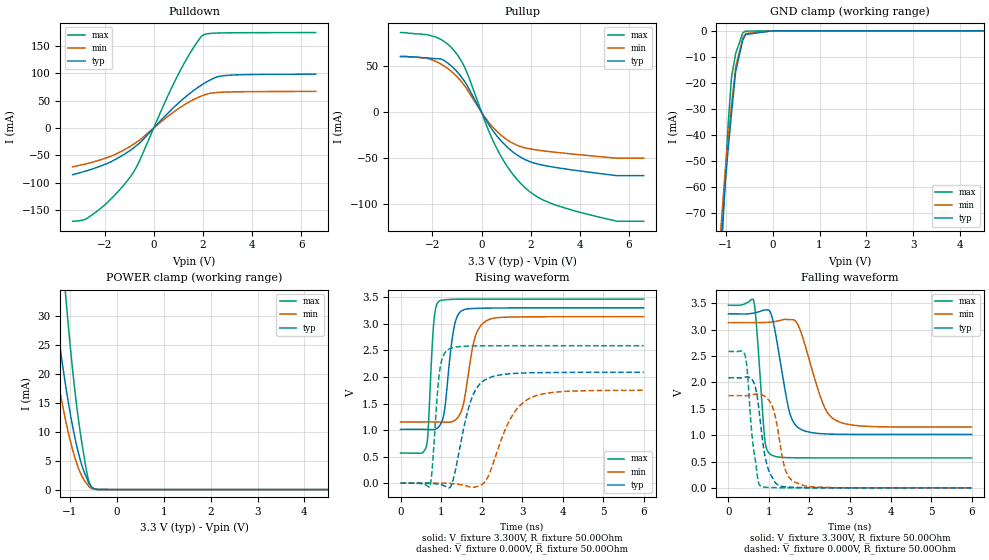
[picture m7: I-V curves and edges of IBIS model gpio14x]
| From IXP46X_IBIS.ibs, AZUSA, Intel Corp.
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[Model]   gpio14x
Model_type   I/O
Vinl = 800.000mV
Vinh = 2.000V
Vmeas = 1.500V
Cref = 0.000F
|   typ   min   max
C_comp   3.000pF   2.700pF   3.300pF
[Voltage Range]   3.300V   3.135V   3.465V
[Temperature Range]   25.0   110.0   -40.0
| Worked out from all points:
|   slope of the pulldown table from 0 to 0.495 V, typ, clamps not added: 21.2 ohm
|   slope of the pullup table from 0 to 0.495 V, typ, clamps not added: 23.4 ohm
|   POWER clamp passes 1 mA (typ) near -0.59 V on its own axis
|   falling waveform, V_fixture 3.300V, R_fixture 50.00Ohm: 20-80 % time 314ps typ, 480ps min, 160ps max; typ from 3.3 V to 1.01 V
|   rising waveform, V_fixture 3.300V, R_fixture 50.00Ohm: 20-80 % time 197ps typ, 269ps min, 114ps max; typ from 1.01 V to 3.3 V
|   rising waveform, V_fixture 0.000V, R_fixture 50.00Ohm: 20-80 % time 396ps typ, 599ps min, 153ps max; typ from 0 V to 2.09 V
|   falling waveform, V_fixture 0.000V, R_fixture 50.00Ohm: 20-80 % time 236ps typ, 261ps min, 185ps max; typ from 2.09 V to 0 V
[Pulldown]
|   Voltage   I(typ)   I(min)   I(max)
-3.3V     -85.26mA   -70.8mA    -170.3mA
-2.8V     -79.09mA   -65.87mA   -166.9mA
-2.265V   -71.22mA   -59.42mA   -150.5mA
-1.585V   -57.94mA   -48.61mA   -122.4mA
-920mV    -39.75mA   -32.53mA   -87.22mA
-600mV    -28.51mA   -22.88mA   -62.16mA
370mV     17.69mA    13.98mA    38.37mA
940mV     42.72mA    33.25mA    92.55mA
1.535V    65.34mA    49.72mA    140.7mA
1.99V     79.66mA    59.11mA    169mA
2.875V    95.55mA    65.49mA    173.5mA
6.595V    98.21mA    66.77mA    174.1mA
[GND Clamp]
|   Voltage   I(typ)   I(min)   I(max)
-3.3V     -1.837A    -1.782A    -2.189A
-1.105V   -83.62mA   -76.71mA   -91.97mA
-1.01V    -58.95mA   -53.8mA    -56.61mA
-950mV    -46.12mA   -41.91mA   -36.62mA
-875mV    -31.66mA   -28.69mA   -17.73mA
-785mV    -15.53mA   -13.65mA   -8.617mA
-635mV    -3.543mA   -2.725mA   -731.7uA
-575mV    -1.513mA   -1.109mA   -135.3uA
0V        -56.84nA   -17.58nA   -65.5pA
6.595V    0A         0A         0A
[Pullup]
|   Voltage   I(typ)   I(min)   I(max)
-3.3V     60.91mA    60.82mA    86.88mA
-1.9V     58.57mA    55.85mA    82.23mA
-1.595V   57.58mA    51.65mA    78.43mA
-1.065V   46.2mA     40.54mA    65.46mA
-630mV    31.07mA    26.68mA    45.51mA
215mV     -9.969mA   -8.214mA   -15.26mA
695mV     -27.97mA   -22.52mA   -43.14mA
1.25V     -42.58mA   -33.21mA   -66.64mA
1.945V    -53.38mA   -39.58mA   -85.97mA
3.84V     -63.17mA   -45.67mA   -107.6mA
5.5V      -68.82mA   -49.81mA   -118.4mA
6.595V    -68.82mA   -49.81mA   -118.5mA
[POWER Clamp]
|   Voltage   I(typ)   I(min)   I(max)
-3.3V     221.1mA    178.3mA    361mA
-1.525V   46.2mA     33.39mA    83.16mA
-1.345V   33.35mA    23.47mA    60.95mA
-1.205V   24.49mA    16.77mA    45.32mA
-1.085V   17.79mA    11.8mA     33.27mA
-950mV    11.36mA    7.178mA    21.48mA
-815mV    6.277mA    3.686mA    12.04mA
-640mV    2mA        1.037mA    3.043mA
-595mV    1.12mA     542.7uA    1.52mA
-540mV    479.4uA    207uA      465.4uA
-390mV    28.44uA    11.22uA    5.344uA
6.595V    0A         0A         0A
[Ramp]
R_load = 50.00Ohm
|   typ   min   max
dV/dt_r   1.253V/394.685ps   1.050V/598.278ps   1.553V/152.725ps
dV/dt_f   1.372V/313.732ps   1.189V/479.440ps   1.738V/159.382ps
[Falling Waveform]
V_fixture = 3.300V
V_fixture_min = 3.135V
V_fixture_max = 3.465V
R_fixture = 50.00Ohm
|   Time   V(typ)   V(min)   V(max)
0s        3.3V       3.135V     3.465V
620ps     3.316V     3.134V     3.559V
690ps     3.328V     3.135V     3.097V
900ps     3.375V     3.139V     898.7mV
1.05ns    3.304V     3.145V     629mV
1.49ns    1.488V     3.194V     572.7mV
1.76ns    1.124V     3.015V     570.1mV
2.35ns    1.025V     1.564V     568.1mV
2.66ns    1.018V     1.278V     568mV
6ns       1.014V     1.153V     568mV
[Rising Waveform]
V_fixture = 3.300V
V_fixture_min = 3.135V
V_fixture_max = 3.465V
R_fixture = 50.00Ohm
|   Time   V(typ)   V(min)   V(max)
0s        1.014V     1.153V     568mV
640ps     1.011V     1.154V     698.2mV
820ps     1.01V      1.153V     3.02V
960ps     1.076V     1.15V      3.431V
1.09ns    1.394V     1.147V     3.452V
1.31ns    2.889V     1.169V     3.462V
1.52ns    3.251V     1.399V     3.464V
1.82ns    3.289V     2.695V     3.465V
2.12ns    3.295V     3.057V     3.465V
6ns       3.3V       3.135V     3.465V
[Rising Waveform]
V_fixture = 0.000V
V_fixture_min = 0.000V
V_fixture_max = 0.000V
R_fixture = 50.00Ohm
|   Time   V(typ)   V(min)   V(max)
0s        824.2nV    300.2nV    -3.119nV
720ps     -80.53uV   180.9uV    -68.76mV
780ps     -2.64mV    387.5uV    258.1mV
970ps     -23.76mV   678.4uV    2.136V
1.19ns    -87.64mV   -2.451mV   2.523V
1.74ns    1.562V     -78.05mV   2.584V
2.09ns    1.947V     31.19mV    2.587V
2.68ns    2.059V     1.166V     2.588V
3.12ns    2.077V     1.57V      2.588V
6ns       2.088V     1.75V      2.588V
[Falling Waveform]
V_fixture = 0.000V
V_fixture_min = 0.000V
V_fixture_max = 0.000V
R_fixture = 50.00Ohm
|   Time   V(typ)   V(min)   V(max)
0s        2.088V     1.75V      2.588V
420ps     2.102V     1.748V     2.484V
610ps     2.023V     1.771V     799.4mV
730ps     1.624V     1.779V     142.6mV
800ps     1.164V     1.771V     30.48mV
910ps     574.6mV    1.73V      11.65mV
1.04ns    250.5mV    1.613V     6.556mV
1.4ns     19.9mV     354.5mV    1.408mV
1.63ns    9.471mV    111.7mV    350.7uV
6ns       824.2nV    300.2nV    -3.119nV
